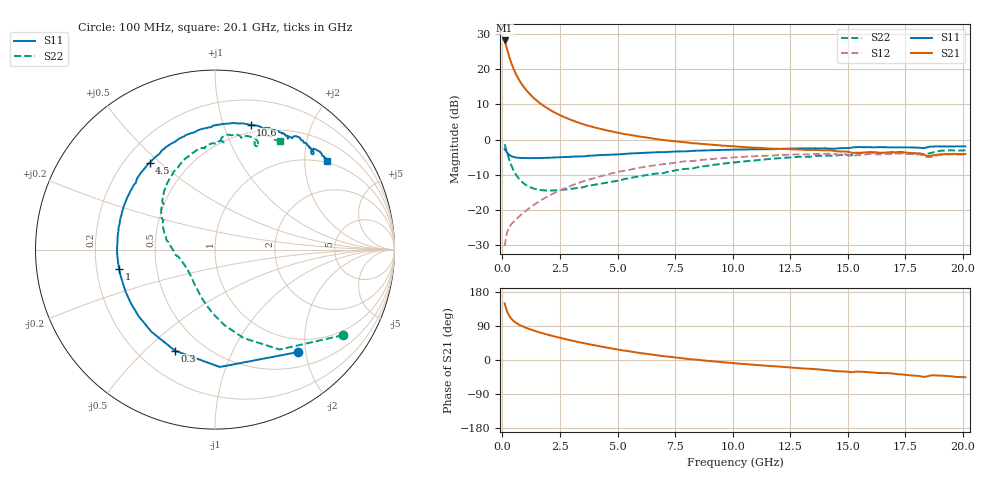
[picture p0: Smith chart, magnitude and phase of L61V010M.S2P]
!  Infineon Technologies AG
! BFR380L3 , PF131585-7, No.6, Th 09.10.01, soldered on pcb-board, measured with PP GSG850
!  Vce=1.0 V,  Ic=10.0 mA
! Common Emitter S-Parameters:  15. November 2001
#  GHz  S  MA  R  50
! f  S11  S21  S12  S22
! GHz  Mag  Ang  Mag  Ang  Mag  Ang  Mag  Ang
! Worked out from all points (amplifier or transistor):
!   201 points, 100 MHz to 20.1 GHz, reference 50 ohm
!   highest |S21| = 28.1 dB at 100 MHz (marker M1)
!   |S21| within 3 dB of that: start of sweep to 228.6 MHz
!   unconditionally stable (mu >= 1): 1.723 GHz to 5.024 GHz; 18.36 GHz to 18.48 GHz
!   at 3.4 GHz: K = 1.03, MAG = 7.2 dB, |S12| = -12.1 dB
!   at 10.1 GHz: K = 0.97, MSG = 1.5 dB, |S12| = -5.0 dB
!   at 20.1 GHz: K = 0.99, MSG = 0.1 dB, |S12| = -4.2 dB
!   S11 on the Smith chart (normalised r, x): 100 MHz: 0.75, -1.86; 300 MHz: 0.35, -0.62; 1 GHz: 0.30, -0.09; 4.5 GHz: 0.30, +0.46; 10.6 GHz: 0.42, +1.23; 20.1 GHz: 0.94, +2.58
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0.1  0.7347 -51.0  25.45 149.5  0.03069 65.7  0.8578 -33.8
0.2  0.6545 -87.6  19.42 129.0  0.04762 53.8  0.663 -57.1
0.3  0.6057 -111.6  14.96 116.6  0.05727 48.5  0.5176 -72.2
0.4  0.5788 -127.7  11.95 108.4  0.06351 46.4  0.4226 -83.1
0.5  0.5645 -139.0  9.874 102.5  0.06885 46.4  0.3589 -91.5
0.6  0.5558 -147.6  8.388 98.0  0.07428 47.2  0.3152 -98.4
0.7  0.5507 -154.4  7.288 94.2  0.07948 48.2  0.2833 -104.4
0.8  0.5465 -160.0  6.431 90.9  0.08475 49.4  0.26 -109.6
1  0.5454 -168.8  5.215 85.6  0.09603 51.5  0.2293 -118.6
1.2  0.5445 -175.7  4.385 81.0  0.1079 52.9  0.2113 -125.9
1.4  0.5457 178.8  3.789 77.0  0.1201 54.1  0.1999 -132.2
1.6  0.5465 173.7  3.342 73.2  0.1325 54.8  0.1936 -137.6
1.9  0.5508 167.0  2.851 68.0  0.1516 55.2  0.1893 -144.6
2.6  0.5624 154.3  2.142 57.1  0.1967 54.2  0.1933 -157.5
3.5  0.5772 140.3  1.653 44.8  0.2549 50.6  0.2094 -169.7
4.5  0.6053 127.1  1.356 33.1  0.3164 45.2  0.2438 177.1
6.8  0.6609 102.3  1.005 11.6  0.4405 30.3  0.3312 151.1
10.1  0.7206 77.4  0.7948 -8.7  0.5593 9.1  0.4751 121.3
10.6  0.7229 74.1  0.7776 -11.2  0.5726 5.9  0.4952 116.9
13.5  0.7465 59.9  0.7131 -23.9  0.6202 -11.2  0.5786 95.0
16.8  0.776 47.7  0.6566 -34.9  0.6226 -26.7  0.6553 74.9
20.1  0.7986 38.3  0.6229 -45.5  0.6142 -40.0  0.7025 59.2
